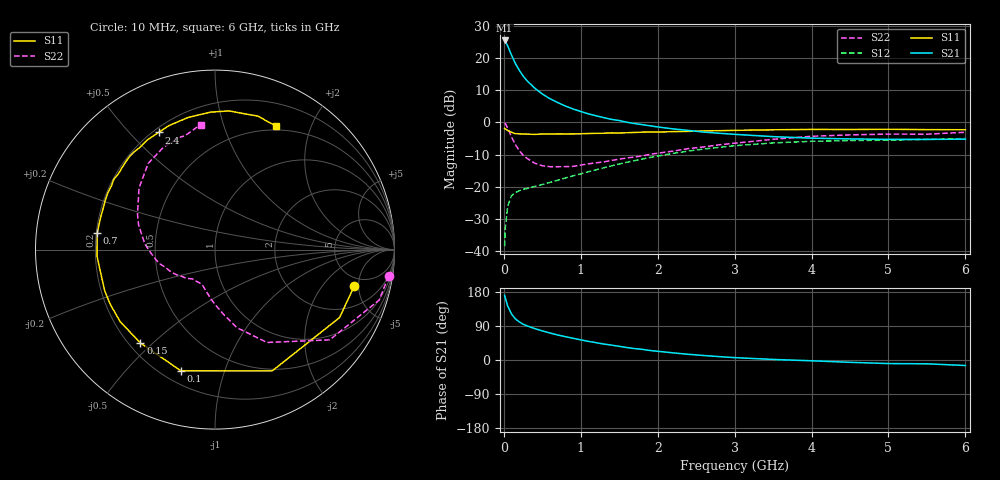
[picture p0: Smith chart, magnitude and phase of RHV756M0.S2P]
! SIEMENS Small Signal Semiconductors
! BFR106
! Si NPN RF Bipolar Junction Transistor in SOT23
! VCE = 0.75 V  IC = 6 mA
! Common Emitter S-Parameters:  August  1996
# GHz  S  MA  R  50
!  f  S11  S21  S12  S22
! GHz  MAG  ANG  MAG  ANG  MAG  ANG  MAG  ANG
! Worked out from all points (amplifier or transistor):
!   36 points, 10 MHz to 6 GHz, reference 50 ohm
!   highest |S21| = 25.5 dB at 10 MHz (marker M1)
!   |S21| within 3 dB of that: start of sweep to 72.73 MHz
!   unconditionally stable (mu >= 1): 549.5 MHz to end of sweep
!   at 250 MHz: K = 0.57, MSG = 17.6 dB, |S12| = -20.8 dB
!   at 1.4 GHz: K = 1.17, MAG = 4.7 dB, |S12| = -13.5 dB
!   at 6 GHz: K = 1.03, MAG = -1.2 dB, |S12| = -5.0 dB
!   S11 on the Smith chart (normalised r, x): 10 MHz: 3.92, -4.45; 100 MHz: 0.27, -0.72; 150 MHz: 0.24, -0.46; 700 MHz: 0.20, +0.07; 2.4 GHz: 0.22, +0.61; 6 GHz: 0.45, +1.52
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0.01  0.8021 -14.6  18.75 170.9  0.0119 84.0  0.9787 -8.7
0.02  0.7907 -28.6  18.28 163.4  0.0234 75.6  0.9567 -17.1
0.05  0.7471 -64.7  15.42 142.5  0.0498 58.3  0.8132 -38.2
0.1  0.7015 -105.7  11.09 121.4  0.0726 43.1  0.5927 -60.8
0.15  0.666 -128.6  8.206 108.5  0.0813 35.8  0.451 -74.4
0.2  0.6636 -142.8  6.473 100.7  0.0863 33.7  0.3657 -82.3
0.25  0.6585 -152.5  5.262 94.6  0.0908 32.8  0.309 -89.4
0.3  0.656 -159.4  4.456 90.2  0.0936 33.7  0.2766 -94.6
0.4  0.6505 -169.4  3.415 83.0  0.101 35.6  0.2326 -103.0
0.5  0.658 -176.6  2.759 76.8  0.1081 37.9  0.2115 -109.0
0.6  0.6574 177.1  2.328 71.2  0.1166 40.8  0.2046 -114.1
0.7  0.6623 172.0  2.032 66.0  0.1259 43.2  0.2046 -119.4
0.9  0.6621 163.6  1.614 57.3  0.1474 46.8  0.2069 -128.2
1.1  0.6708 155.5  1.355 49.1  0.171 49.0  0.2265 -135.7
1.3  0.6772 148.3  1.183 42.1  0.1969 49.7  0.2433 -143.5
1.6  0.6895 138.9  1.002 32.9  0.2398 49.2  0.2793 -154.9
2.2  0.7183 121.5  0.791 18.8  0.3293 43.1  0.3575 -176.9
2.4  0.7246 115.7  0.749 15.0  0.3585 40.2  0.3911 175.6
3.5  0.7662 91.9  0.6 1.5  0.4792 21.6  0.5453 140.9
4.5  0.7743 77.8  0.553 -6.1  0.5207 6.0  0.639 116.6
5.5  0.7705 67.2  0.543 -10.1  0.5448 -3.2  0.6553 104.9
6  0.7676 63.6  0.548 -14.5  0.5604 -9.7  0.7012 96.6
